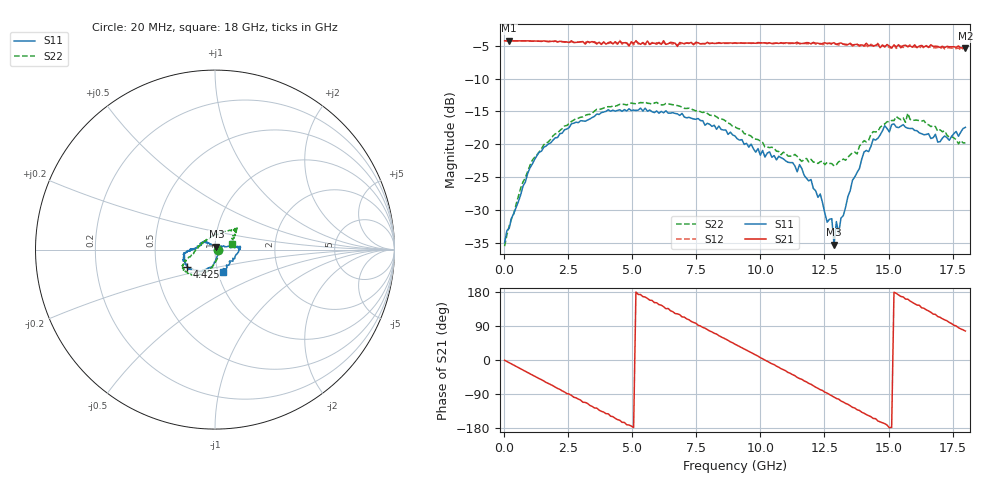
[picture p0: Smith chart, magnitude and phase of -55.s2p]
!Agilent Technologies,N5230A,US43500223,A.07.50.48
!Agilent N5230A: A.07.50.48
!Date: Saturday, January 16, 2016 12:43:53
!Correction: S11(Full 2 Port(1,2))
!S21(Full 2 Port(1,2))
!S12(Full 2 Port(1,2))
!S22(Full 2 Port(1,2))
!S2P File: Measurements: S11, S21, S12, S22:
# Hz S  dB  R 50
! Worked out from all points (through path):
!   201 points, 20 MHz to 18 GHz, reference 50 ohm
!   highest |S21| = -4.22 dB at 199.8 MHz (marker M1); lowest = -5.4 dB at 18 GHz (marker M2)
!   group delay of S21, straight-line fit = 99.1 ps
!   lowest |S11| = -35.3 dB at 12.88 GHz (marker M3), VSWR 1.03, Z = 50.7 + j1.57 ohm
!   |S11| at or under -10 dB: start of sweep to end of sweep
!   |S22| runs from -35.5 to -13.6 dB; largest |S21 - S12| = 0.071
!   S11 on the Smith chart (normalised r, x): 20 MHz: 1.04, -0.00; 4.425 GHz: 0.72, -0.14; 18 GHz: 1.06, -0.27
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2e7  -35.02 -3.8  -4.22 -0.7  -4.23 -0.8  -35.55 -5.6
1.998e8  -32.81 -33.5  -4.22 -7.2  -4.23 -7.3  -32.46 -35.3
1.3685e9  -21.21 -96.0  -4.30 -49.2  -4.29 -49.5  -21.19 -96.3
2.1776e9  -18.39 -113.3  -4.30 -77.6  -4.35 -78.4  -17.90 -108.7
3.0766e9  -16.44 -127.4  -4.35 -111.5  -4.38 -111.2  -15.82 -122.2
4.4251e9  -14.86 -148.4  -4.66 -157.3  -4.75 -157.8  -14.09 -138.0
5.1443e9  -14.85 -156.7  -4.26 179.3  -4.20 177.8  -13.84 -144.7
6.0433e9  -15.28 -169.7  -4.48 146.2  -4.58 143.1  -13.87 -149.8
7.4817e9  -16.20 -176.5  -4.45 97.0  -4.64 93.5  -14.92 -157.6
9.01e9  -18.74 176.5  -4.56 41.7  -4.59 38.9  -17.36 -166.5
1.06282e10  -22.39 153.5  -4.58 -16.3  -4.56 -19.1  -21.07 168.8
1.15272e10  -23.11 141.7  -4.68 -48.9  -4.59 -52.9  -22.29 150.2
1.20666e10  -26.74 131.6  -4.47 -68.1  -4.54 -71.8  -22.73 137.9
1.2606e10  -31.89 118.9  -4.67 -87.4  -4.62 -91.5  -22.77 127.2
1.27858e10  -31.36 99.8  -4.63 -94.4  -4.77 -98.2  -22.95 120.1
1.28757e10  -35.31 64.0  -4.52 -97.8  -4.68 -101.3  -23.31 118.4
1.29656e10  -31.79 75.8  -4.79 -101.6  -4.73 -106.2  -23.11 116.0
1.30555e10  -33.60 67.8  -4.63 -103.3  -4.88 -108.3  -22.66 108.0
1.40444e10  -21.20 12.7  -4.97 -140.5  -5.07 -143.6  -19.45 70.2
1.50333e10  -18.13 5.9  -5.06 -178.7  -5.27 178.7  -16.56 50.3
1.65616e10  -18.39 -25.0  -5.25 129.6  -5.14 122.9  -17.04 38.3
1.8e10  -17.43 -69.5  -5.39 76.4  -5.47 69.3  -19.79 18.4
